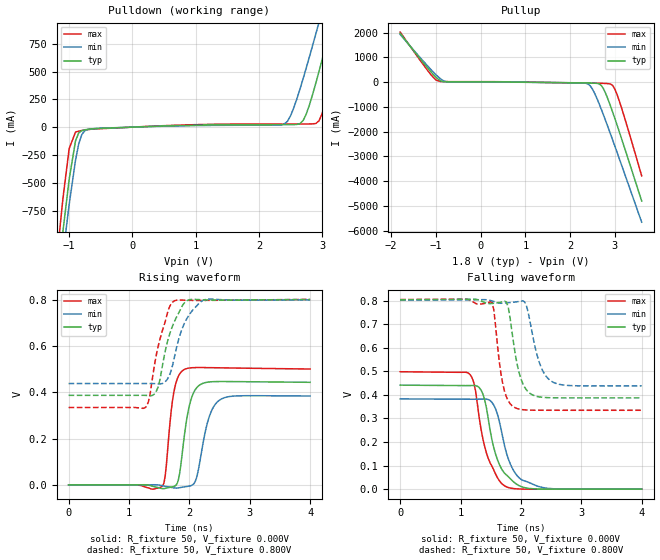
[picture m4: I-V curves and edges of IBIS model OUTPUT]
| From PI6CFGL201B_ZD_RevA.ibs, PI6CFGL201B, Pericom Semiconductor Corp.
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|   Model OUTPUT
[Model]  OUTPUT
Model_type Output
Vref = 1.80V
Vmeas = 0.95V
C_comp   3.770pF   3.760pF   3.780pF
[Voltage Range]   1.8000V   1.6200V   1.9800V
[POWER Clamp Reference]  1.8000V   1.6200V   1.9800V
[GND Clamp Reference]   0.0000V   0.0000V   0.0000V
[Pullup Reference]   1.8000V   1.6200V   1.9800V
[Pulldown Reference]   0.0000V   0.0000V   0.0000V
[Temperature Range]   25   85   -40
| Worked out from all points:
|   slope of the pulldown table from 0 to 0.27 V, typ, clamps not added: 45.2 ohm
|   slope of the pullup table from 0 to 0.27 V, typ, clamps not added: 121 ohm
|   rising waveform, R_fixture 50, V_fixture 0.000V: 20-80 % time 152ps typ, 189ps min, 119ps max; typ from 0 V to 0.443 V
|   falling waveform, R_fixture 50, V_fixture 0.000V: 20-80 % time 253ps typ, 261ps min, 256ps max; typ from 0.441 V to 0 V
|   rising waveform, R_fixture 50, V_fixture 0.800V: 20-80 % time 251ps typ, 263ps min, 233ps max; typ from 0.387 V to 0.802 V
|   falling waveform, R_fixture 50, V_fixture 0.800V: 20-80 % time 174ps typ, 209ps min, 144ps max; typ from 0.803 V to 0.387 V
[Pulldown]
|Voltage   I(typ)   I(min)   I(max)
-1.8V     -4.798A    -4.74A     -4.904A
-1.2V     -1.464A    -1.646A    -1.21A
-1.1V     -943.8mA   -1.157A    -648.2mA
-1V       -468.7mA   -695.8mA   -193mA
-900mV    -124.4mA   -298.5mA   -44.89mA
-700mV    -19.59mA   -20.13mA   -21.59mA
2.4V      22.34mA    27.55mA    28.36mA
2.7V      60.52mA    439.2mA    28.53mA
2.9V      397.2mA    840mA      33.13mA
3.15V     942.1mA    1.364A     442.3mA
3.35V     1.398A     1.791A     931.4mA
3.6V      1.975A     2.325A     1.567A
[Pullup]
|Voltage   I(typ)   I(min)   I(max)
-1.8V     1.97A      1.929A     2.025A
-1.1V     391.9mA    487.9mA    278.3mA
-900mV    55.2mA     138.9mA    26.38mA
-700mV    17.17mA    12.9mA     24.1mA
2.4V      -31.19mA   -71.25mA   -33.8mA
2.5V      -36.32mA   -279.7mA   -35.84mA
2.7V      -138mA     -1.106A    -43.69mA
2.8V      -474.8mA   -1.584A    -52.41mA
2.9V      -946.7mA   -2.078A    -71.33mA
3V        -1.466A    -2.582A    -279.3mA
3.2V      -2.557A    -3.602A    -1.329A
3.6V      -4.798A    -5.655A    -3.782A
[Rising Waveform]
R_fixture = 50
V_fixture = 0.000V
V_fixture_min = 0.000V
V_fixture_max = 0.000V
|   Time   V(typ)   V(min)   V(max)
0s        64.77uV    70.65uV    56.18uV
1.56ns    -16.73mV   -4.226mV   -3.648mV
1.6ns     -15.49mV   -6.442mV   38.47mV
1.74ns    -7.272mV   -12.98mV   396.1mV
1.82ns    23.34mV    -13.36mV   470.7mV
1.92ns    218mV      -8.735mV   499.2mV
2.1ns     412.4mV    15.94mV    507mV
2.32ns    444.6mV    286.8mV    506.8mV
2.5ns     446.7mV    366.3mV    506.1mV
4ns       443.4mV    384.2mV    500.8mV
[Falling Waveform]
R_fixture = 50
V_fixture = 0.000V
V_fixture_min = 0.000V
V_fixture_max = 0.000V
|   Time   V(typ)   V(min)   V(max)
0s        441.2mV    382.9mV    498mV
1.16ns    439.4mV    381.4mV    485.5mV
1.25ns    439.3mV    381.4mV    414.7mV
1.37ns    403.7mV    382.1mV    213.4mV
1.52ns    209.4mV    368.3mV    97.12mV
1.61ns    125.9mV    318.8mV    49.17mV
1.76ns    60.34mV    153.7mV    10.09mV
1.97ns    14.89mV    48.34mV    932uV
2.33ns    550.8uV    8.924mV    106.9uV
4ns       82.65uV    91.81uV    69.13uV
[Rising Waveform]
R_fixture = 50
V_fixture = 0.800V
V_fixture_min = 0.800V
V_fixture_max = 0.800V
|   Time   V(typ)   V(min)   V(max)
0s        387.1mV    438mV      334.6mV
1.28ns    386.8mV    438mV      336.8mV
1.34ns    385.3mV    437.9mV    378.9mV
1.48ns    421.7mV    436.9mV    595.2mV
1.64ns    621.8mV    458.6mV    745.4mV
1.76ns    710.5mV    560.7mV    796.5mV
1.84ns    751.9mV    644.4mV    799.2mV
1.94ns    792.7mV    710.2mV    798.4mV
2.24ns    799.9mV    799.3mV    797.6mV
4ns       801.6mV    799.9mV    801.8mV
[Falling Waveform]
R_fixture = 50
V_fixture = 0.800V
V_fixture_min = 0.800V
V_fixture_max = 0.800V
|   Time   V(typ)   V(min)   V(max)
0s        803.5mV    801.5mV    803.9mV
1.52ns    787.6mV    798.4mV    793.2mV
1.55ns    788.3mV    796.1mV    762.2mV
1.67ns    793.1mV    788.3mV    488.6mV
1.76ns    793.9mV    789.9mV    391.3mV
1.91ns    567.3mV    794mV      344.7mV
2.09ns    421.6mV    779.4mV    335.9mV
2.3ns     391.5mV    540.8mV    334.8mV
2.51ns    387.6mV    457mV      334.7mV
4ns       387.1mV    438mV      334.7mV
[Ramp]
| variable   typ   min   max
dV/dt_r  0.2673/153.82p   0.2309/189.77p   0.3024/122.05p
dV/dt_f  0.2505/173.64p   0.2186/207.93p   0.2823/141.83p
R_load = 50.0000
